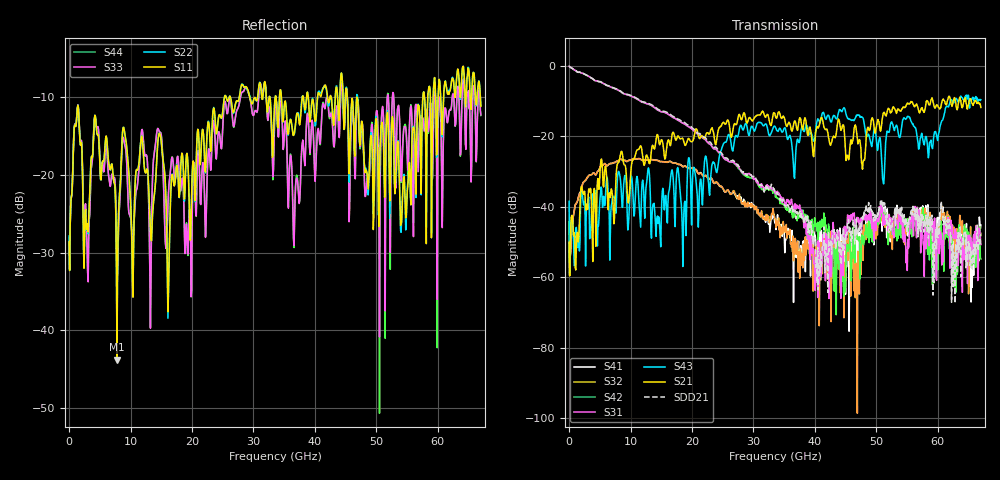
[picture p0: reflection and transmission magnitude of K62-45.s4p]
!Agilent Technologies,N5247A,US50470101,A.10.25.02
!Agilent N5247A: A.10.25.02
!Date: Tuesday, May 12, 2015 13:42:52
!Correction: Sdd11(Full 4 Port(1,2,3,4))
!Sdc11(Full 4 Port(1,2,3,4))
!Sdd12(Full 4 Port(1,2,3,4))
!Sdc12(Full 4 Port(1,2,3,4))
!Scd11(Full 4 Port(1,2,3,4))
!Scc11(Full 4 Port(1,2,3,4))
!Scd12(Full 4 Port(1,2,3,4))
!Scc12(Full 4 Port(1,2,3,4))
!Sdd21(Full 4 Port(1,2,3,4))
!Sdc21(Full 4 Port(1,2,3,4))
!Sdd22(Full 4 Port(1,2,3,4))
!Sdc22(Full 4 Port(1,2,3,4))
!Scd21(Full 4 Port(1,2,3,4))
!Scc21(Full 4 Port(1,2,3,4))
!Scd22(Full 4 Port(1,2,3,4))
!Scc22(Full 4 Port(1,2,3,4))
!Balanced Topology: BBAL
!S4P File: Measurements: <Sdd11,Sdc11,Sdd12,Sdc12>,
!<Scd11,Scc11,Scd12,Scc12>,
!<Sdd21,Sdc21,Sdd22,Sdc22>,
!<Scd21,Scc21,Scd22,Scc22>:
# Hz S  dB  R 50
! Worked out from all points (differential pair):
!   801 points, 10 MHz to 67 GHz, reference 50 ohm
!   strongest paths, dB at 10 MHz, 16.76 GHz, 33.51 GHz, 50.25 GHz, 67 GHz:
!     S21: -50.1, -19.4, -13.7, -15.2, -11.8
!     S43: -38.4, -29.5, -17.2, -23.6, -9.6
!     S31: -0.1, -14.5, -36.1, -43.2, -50.7
!     S42: -0.1, -14.4, -36.3, -45.1, -54.8
!     S32: -52.2, -27.4, -43.4, -44.2, -47.4
!     S41: -44.2, -27.4, -44.6, -43.9, -45.1
!   taken as a pair (ports 1,2 in; 3,4 out), SDD21 dB: 0.0, -14.1, -35.9, -41.7, -47.7
!   lowest |S11| = -43.8 dB at 7.798 GHz (marker M1), VSWR 1.01, Z = 49.7 - j0.585 ohm
!   |S11| at or under -10 dB: start of sweep to 25.29 GHz; 34.54 GHz to 37.94 GHz (3.397 GHz wide, 9.37 % of centre); 46.84 GHz to 57.57 GHz (10.73 GHz wide, 20.6 % of centre)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
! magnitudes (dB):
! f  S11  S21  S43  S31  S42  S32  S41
! 10 MHz  -28.6  -50.1  -38.4  -0.1  -0.1  -52.2  -44.2
! 1.266 GHz  -12.4  -48.3  -47.8  -1.6  -1.6  -38.6  -38.7
! 7.798 GHz  -43.8  -28.4  -34.2  -6.7  -6.7  -27.0  -27.0
! 18.77 GHz  -23.1  -22.1  -38.8  -16.4  -16.4  -28.4  -28.4
! 27.98 GHz  -8.7  -15.1  -16.9  -29.8  -30.0  -38.0  -37.2
! 39.95 GHz  -12.6  -22.2  -20.8  -55.2  -43.0  -56.6  -49.5
! 67 GHz  -11.2  -11.8  -9.6  -50.7  -54.8  -47.4  -45.1
